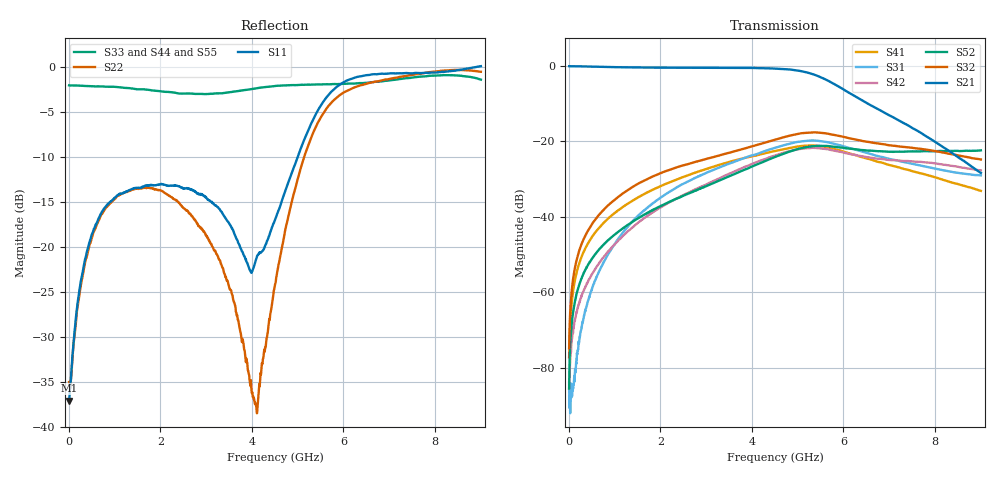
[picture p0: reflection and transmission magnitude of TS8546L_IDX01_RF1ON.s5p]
# GHz S DB R 50
! CMT, SN0916, 25263762, 26.7.0
! Date: 16.07.2026 12:21:22
! Data: Format
! Freq S1.1:dB/Ang S1.2:dB/Ang S1.3:dB/Ang S1.4:dB/Ang S1.5:dB/Ang
!  S2.1:dB/Ang S2.2:dB/Ang S2.3:dB/Ang S2.4:dB/Ang S2.5:dB/Ang
!  S3.1:dB/Ang S3.2:dB/Ang S3.3:dB/Ang S3.4:dB/Ang S3.5:dB/Ang
!  S4.1:dB/Ang S4.2:dB/Ang S4.3:dB/Ang S4.4:dB/Ang S4.5:dB/Ang
!  S5.1:dB/Ang S5.2:dB/Ang S5.3:dB/Ang S5.4:dB/Ang S5.5:dB/Ang
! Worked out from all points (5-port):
!   2001 points, 10 MHz to 9 GHz, reference 50 ohm
!   strongest paths, dB at 10 MHz, 2.257 GHz, 4.505 GHz, 6.753 GHz, 9 GHz:
!     S21: -0.2, -0.6, -0.8, -11.6, -28.4
!     S32: -74.8, -27.4, -19.6, -20.6, -24.9
!     S52: -85.5, -35.7, -24.2, -22.7, -22.5
!     S42: -85.5, -35.8, -23.8, -24.7, -27.7
!     S31: -83.9, -33.0, -21.8, -24.0, -29.1
!     S41: -77.2, -30.6, -22.6, -25.5, -33.2
!   lowest |S11| = -37.1 dB at 10 MHz (marker M1), VSWR 1.03, Z = 51.4 - j0.136 ohm
!   |S11| at or under -10 dB: start of sweep to 5.003 GHz
